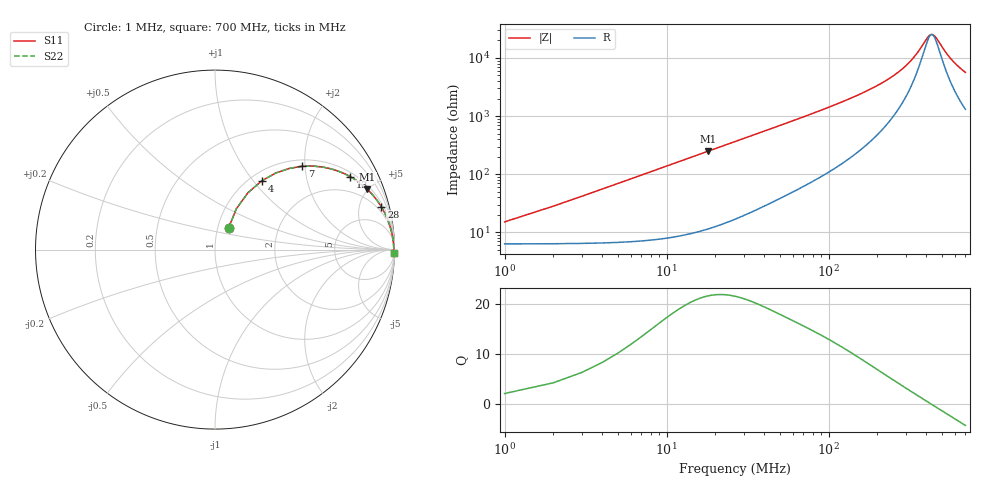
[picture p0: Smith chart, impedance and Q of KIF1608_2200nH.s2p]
# MHz S RI R 50
!Freq ReS11 ImS11 ReS21 ImS21 ReS12 ImS12 ReS22 ImS22
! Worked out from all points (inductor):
!   700 points, 1 MHz to 700 MHz, reference 50 ohm
!   read as one part in series: L = 2.2 uH near 4 MHz
!   highest Q = 21.6 at 18 MHz (marker M1), where L = 2.19 uH
!   self-resonance near 433.9 MHz
!   S11 on the Smith chart (normalised r, x): 1 MHz: 1.13, +0.28; 4 MHz: 1.13, +1.10; 7 MHz: 1.14, +1.93; 13 MHz: 1.18, +3.59; 28 MHz: 1.36, +7.70; 700 MHz: open
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1  0.0753 0.12  0.9247 -0.12  0.9247 -0.12  0.0753 0.12
4  0.2604 0.3831  0.7396 -0.3831  0.7396 -0.3831  0.2604 0.3831
5  0.3394 0.4271  0.6606 -0.4271  0.6606 -0.4271  0.3394 0.4271
7  0.4853 0.4642  0.5147 -0.4642  0.5147 -0.4642  0.4853 0.4642
10  0.6483 0.4495  0.3517 -0.4495  0.3517 -0.4495  0.6483 0.4495
13  0.7524 0.4071  0.2476 -0.4071  0.2476 -0.4071  0.7524 0.4071
18  0.8493 0.3354  0.1507 -0.3354  0.1507 -0.3354  0.8493 0.3354
28  0.9273 0.2374  0.0727 -0.2374  0.0727 -0.2374  0.9273 0.2374
43  0.9642 0.1614  0.0358 -0.1614  0.0358 -0.1614  0.9642 0.1614
62  0.9798 0.1136  0.0202 -0.1136  0.0202 -0.1136  0.9798 0.1136
87  0.9876 0.0806  0.0124 -0.0806  0.0124 -0.0806  0.9876 0.0806
118  0.9916 0.0579  0.00838 -0.0579  0.00838 -0.0579  0.9916 0.0579
234  0.9954 0.0226  0.00463 -0.0226  0.00463 -0.0226  0.9954 0.0226
300  0.9958 0.013  0.00416 -0.013  0.00416 -0.013  0.9958 0.013
351  0.996 0.00736  0.00401 -0.00736  0.00401 -0.00736  0.996 0.00736
401  0.996 0.00272  0.00395 -0.00272  0.00395 -0.00272  0.996 0.00272
421  0.9961 0.00104  0.00394 -0.00104  0.00394 -0.00104  0.9961 0.00104
442  0.9961 -0.000636  0.00395 0.000636  0.00395 0.000636  0.9961 -0.000636
467  0.996 -0.00253  0.00396 0.00253  0.00396 0.00253  0.996 -0.00253
527  0.996 -0.00674  0.00402 0.00674  0.00402 0.00674  0.996 -0.00674
584  0.9959 -0.0104  0.00411 0.0104  0.00411 0.0104  0.9959 -0.0104
700  0.9956 -0.0171  0.00439 0.0171  0.00439 0.0171  0.9956 -0.0171
